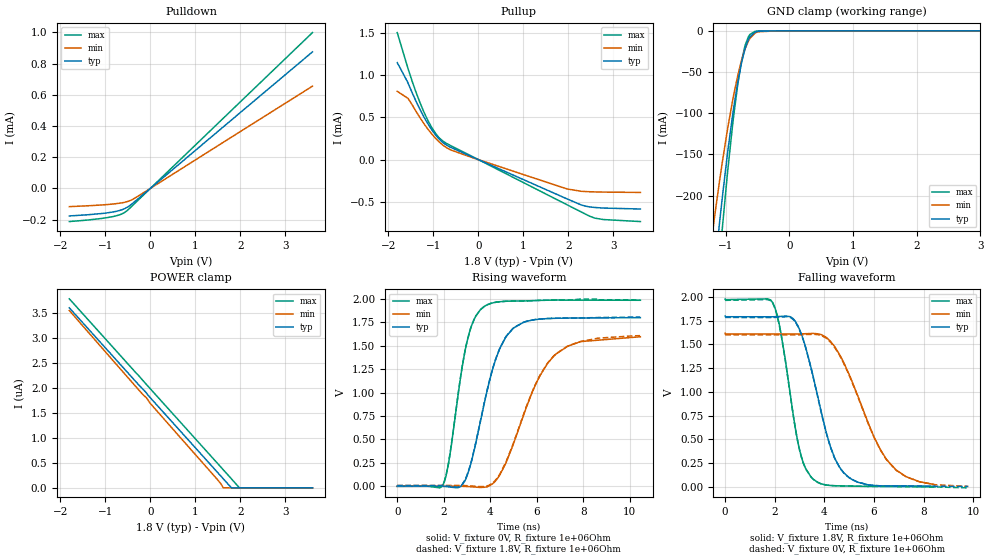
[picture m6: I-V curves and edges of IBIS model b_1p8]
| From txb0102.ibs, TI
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|   b_1p8 Model
[Model]   b_1p8
Model_type   I/O
Polarity   Non-Inverting
Enable   Active-High
Vinl = 0.63
Vinh = 1.17
Vmeas = 0.9
Vref = 0
Cref = 2pF
Rref = 1e6
|   typ   min   max
|   (nom PVT)   (fast PVT)   (slow PVT)
C_comp   1.097e-11   1.083e-11   1.097e-11
[Model spec]
|subparameter
Vinl   0.63   0.567   0.693
Vinh   1.17   1.053   1.287
| Where nom  PVT is Nominal Process, 1.8V, 27C
|   Fast PVT is Strong Process,  1.98V, -40C
|   Slow PVT is Weak Process,   1.62V, 125C
[Voltage Range]   1.8   1.62   1.98
|Junction Temperature
[Temperature Range]   27   125   -40
[Pullup Reference]   1.8   1.62   1.98
[Pulldown Reference]   0   0   0
[Power Clamp Reference]   1.8   1.62   1.98
[GND Clamp Reference]   0   0   0
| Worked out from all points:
|   slope of the pulldown table from 0 to 0.27 V, typ, clamps not added: 4.11 kohm
|   slope of the pullup table from 0 to 0.27 V, typ, clamps not added: 4.22 kohm
|   GND clamp passes 1 mA (typ) near -0.52 V on its own axis
|   falling waveform, V_fixture 1.8V, R_fixture 1e+06Ohm: 20-80 % time 1.05ns typ, 1.58ns min, 723ps max; typ from 1.8 V to 0.003 V
|   rising waveform, V_fixture 0V, R_fixture 1e+06Ohm: 20-80 % time 1.08ns typ, 1.59ns min, 747ps max; typ from 0 V to 1.8 V
|   rising waveform, V_fixture 1.8V, R_fixture 1e+06Ohm: 20-80 % time 1.08ns typ, 1.61ns min, 746ps max; typ from 0.007 V to 1.8 V
|   falling waveform, V_fixture 0V, R_fixture 1e+06Ohm: 20-80 % time 1.05ns typ, 1.6ns min, 726ps max; typ from 1.78 V to 0.001 V
[Pulldown]
|   Voltage   I(typ)   I(min)   I(max)
-1.8V     -176.6uA   -117uA     -212.6uA
-851.4mV  -152.1uA   -100.7uA   -181.8uA
-680.4mV  -141.3uA   -94.84uA   -168.9uA
-531mV    -123.9uA   -86.17uA   -145.6uA
-396mV    -96.14uA   -70.59uA   -110uA
-180mV    -43.84uA   -32.84uA   -49.99uA
3.6V      874.5uA    654.9uA    998.1uA
[GND Clamp]
|   Voltage   I(typ)   I(min)   I(max)
-1.8V     -870.6mA   -666.1mA   -1.052A
-1.183V   -297.2mA   -230.1mA   -358.4mA
-1.095V   -231.7mA   -181.3mA   -276.5mA
-1.057V   -204.4mA   -161mA     -242.3mA
-962.5mV  -143.1mA   -115.2mA   -165.3mA
-875.3mV  -93.62mA   -78.06mA   -103.4mA
-812mV    -62.95mA   -54.67mA   -65.7mA
-754.6mV  -39.79mA   -36.66mA   -38.18mA
-701.1mV  -22.99mA   -23.12mA   -19.45mA
-645.7mV  -11.02mA   -12.76mA   -7.609mA
-538.7mV  -1.54mA    -2.749mA   -582.8uA
3.6V      0A         0A         0A
[Pullup]
|   Voltage   I(typ)   I(min)   I(max)
-1.8V     1.148mA    808.7uA    1.504mA
-1.559V   903.1uA    724.1uA    1.074mA
-1.386V   694.1uA    573.9uA    801.5uA
-1.206V   503.5uA    424.4uA    561uA
-1.024V   345.4uA    297.3uA    371uA
-780.3mV  199.4uA    169.2uA    216.8uA
-180mV    42.6uA     31.82uA    48.98uA
1.955V    -461.6uA   -344.2uA   -530.5uA
2.288V    -537.2uA   -375.4uA   -620.5uA
2.592V    -567.2uA   -382.6uA   -693.4uA
2.776V    -574uA     -384.9uA   -709.8uA
3.6V      -585uA     -388.8uA   -733.7uA
[POWER Clamp]
|   Voltage   I(typ)   I(min)   I(max)
-1.8V     3.601uA    3.547uA    3.78uA
-259.6mV  2.061uA    1.96uA     2.244uA
-89.28mV  1.898uA    1.801uA    2.069uA
50.04mV   1.75uA     1.635uA    1.93uA
1.485V    314.7nA    168.2nA    494.6nA
1.568V    232.3nA    76.48nA    412.2nA
1.617V    183.5nA    0A         363.4nA
1.802V    0A         0A         178.2nA
1.978V    0A         0A         0A
3.6V      0A         0A         0A
[Ramp]
R_load = 1e+06
|   typ   min   max
dV/dt_r   1.07392/1.06557e-09  0.962627/1.5933e-09   1.1886/7.38851e-10
dV/dt_f   1.0774/1.04696e-09   0.969338/1.6057e-09   1.18463/7.1856e-10
[Falling Waveform]
V_fixture = 1.8V
V_fixture_min = 1.62V
V_fixture_max = 1.98V
R_fixture = 1e+06Ohm
|   Time   V(typ)   V(min)   V(max)
0s        1.8V       1.62V      1.98V
1.928ns   1.792V     1.611V     1.937V
2.258ns   1.796V     1.61V      1.606V
3.002ns   1.657V     1.611V     386.4mV
3.562ns   1.146V     1.616V     75.53mV
4.246ns   419.3mV    1.533V     11.82mV
4.974ns   99.39mV    1.198V     5.899mV
6.528ns   6.748mV    279mV      1.164mV
7.296ns   6.038mV    104.5mV    806uV
8.454ns   3.22mV     20.13mV    -3.123mV
[Rising Waveform]
V_fixture = 0V
V_fixture_min = 0V
V_fixture_max = 0V
R_fixture = 1e+06Ohm
|   Time   V(typ)   V(min)   V(max)
0s        52.17nV    14.83uV    28.49nV
1.972ns   -628uV     149.3uV    17.74mV
2.212ns   -5.868mV   468.1uV    249.7mV
3.002ns   110.9mV    -2.189mV   1.542V
3.754ns   896.2mV    -9.903mV   1.92V
4.194ns   1.323V     47.39mV    1.962V
4.708ns   1.606V     267.5mV    1.975V
5.916ns   1.778V     1.065V     1.982V
6.73ns    1.792V     1.388V     1.987V
10.46ns   1.8V       1.596V     1.985V
[Rising Waveform]
V_fixture = 1.8V
V_fixture_min = 1.62V
V_fixture_max = 1.98V
R_fixture = 1e+06Ohm
|   Time   V(typ)   V(min)   V(max)
0s        7.33mV     8.755mV    7.079mV
1.976ns   6.729mV    8.996mV    26.66mV
2.212ns   1.57mV     9.308mV    256.3mV
3ns       116.8mV    6.692mV    1.543V
3.754ns   902.1mV    -1.017mV   1.921V
4.192ns   1.325V     55.67mV    1.962V
4.706ns   1.607V     275.1mV    1.975V
5.914ns   1.778V     1.07V      1.982V
6.724ns   1.793V     1.389V     1.987V
10.45ns   1.804V     1.607V     1.986V
[Falling Waveform]
V_fixture = 0V
V_fixture_min = 0V
V_fixture_max = 0V
R_fixture = 1e+06Ohm
|   Time   V(typ)   V(min)   V(max)
0s        1.785V     1.602V     1.966V
1.928ns   1.784V     1.602V     1.93V
2.258ns   1.789V     1.601V     1.599V
3ns       1.65V      1.602V     385mV
3.562ns   1.139V     1.607V     74.8mV
4.242ns   418.3mV    1.526V     11.79mV
4.972ns   98.81mV    1.191V     5.831mV
5.996ns   11.76mV    522mV      1.791mV
6.884ns   6.376mV    174.5mV    1.062mV
9.8ns     1.172mV    2.905mV    -13.16mV
